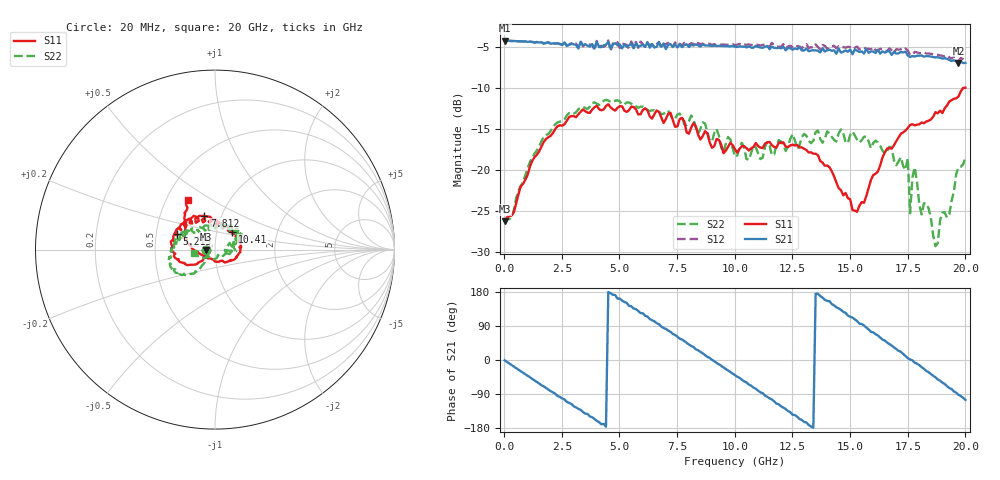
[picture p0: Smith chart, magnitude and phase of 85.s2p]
!Agilent Technologies,N5230A,US43500223,A.07.50.48
!Agilent N5230A: A.07.50.48
!Date: Tuesday, September 15, 2015 19:49:33
!Correction: S11(Full 2 Port(1,2))
!S21(Full 2 Port(1,2))
!S12(Full 2 Port(1,2))
!S22(Full 2 Port(1,2))
!S2P File: Measurements: S11, S21, S12, S22:
# Hz S  RI  R 50
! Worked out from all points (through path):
!   201 points, 20 MHz to 20 GHz, reference 50 ohm
!   highest |S21| = -4.26 dB at 20 MHz (marker M1); lowest = -7.0 dB at 19.7 GHz (marker M2)
!   group delay of S21, straight-line fit = 114 ps
!   lowest |S11| = -26.3 dB at 20 MHz (marker M3), VSWR 1.10, Z = 45.4 + j0.0423 ohm
!   |S11| at or under -10 dB: start of sweep to end of sweep
!   |S22| runs from -29.3 to -11.5 dB; largest |S21 - S12| = 0.062
!   S11 on the Smith chart (normalised r, x): 20 MHz: 0.91, +0.00; 5.215 GHz: 0.64, +0.12; 7.812 GHz: 0.83, +0.33; 10.41 GHz: 1.18, +0.24; 20 GHz: 0.64, +0.40
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2e7  -0.0484 0.000465  0.6122 -0.00901  0.6126 -0.00941  -0.0478 -0.00313
1.9181e9  -0.1337 -0.0838  0.1271 -0.5851  0.1297 -0.5817  -0.1095 -0.1234
3.4166e9  -0.2297 -0.0372  -0.4203 -0.3892  -0.4201 -0.3742  -0.2037 -0.1293
4.5155e9  -0.2462 0.0461  -0.6015 0.00789  -0.6132 0.00783  -0.2521 -0.0782
5.2148e9  -0.2118 0.0861  -0.5168 0.262  -0.531 0.2383  -0.2455 -0.0443
6.7133e9  -0.1446 0.172  -0.046 0.5941  -0.0574 0.5985  -0.2191 0.0535
7.8122e9  -0.0586 0.1878  0.3681 0.4403  0.3802 0.4551  -0.1696 0.0836
8.9111e9  0.0209 0.1454  0.5682 0.0533  0.581 0.0729  -0.1168 0.0936
1.001e10  0.0811 0.1054  0.4306 -0.361  0.4548 -0.3491  -0.0526 0.1075
1.04096e10  0.0958 0.1007  0.3137 -0.4684  0.3455 -0.4647  -0.03 0.1323
1.16084e10  0.1341 0.0438  -0.1388 -0.5445  -0.1305 -0.578  0.0329 0.1181
1.34066e10  0.1181 -0.0414  -0.5341 -0.0126  -0.5484 -0.056  0.1037 0.1085
1.53047e10  -0.0228 -0.0505  -0.1176 0.5181  -0.1344 0.5467  0.1361 0.0679
1.67033e10  -0.1339 0.0177  0.3907 0.3563  0.3987 0.3765  0.1261 0.0556
1.75025e10  -0.1695 0.0589  0.4945 0.0423  0.5303 0.0567  0.1169 -0.00961
1.76024e10  -0.1732 0.0713  0.4859 0.0109  0.5004 0.0204  0.0541 -0.00328
1.78022e10  -0.1702 0.0754  0.4861 -0.0599  0.5215 -0.0221  0.1032 0.00367
1.81019e10  -0.1671 0.0985  0.4696 -0.1618  0.4927 -0.1533  0.0532 -0.00274
1.84016e10  -0.1652 0.1103  0.417 -0.2614  0.4377 -0.2627  0.0476 -0.0336
1.87013e10  -0.1754 0.1393  0.3388 -0.3443  0.3591 -0.3509  0.015 -0.0307
1.97003e10  -0.1534 0.2332  -0.0132 -0.4461  0.00365 -0.4583  -0.0972 -0.0348
2e10  -0.1516 0.2773  -0.1179 -0.4315  -0.108 -0.4477  -0.1168 -0.0213
